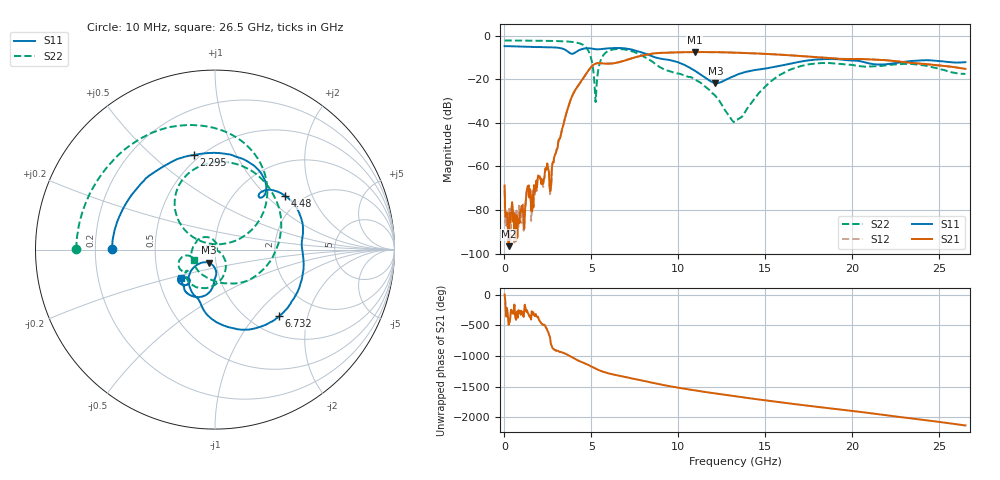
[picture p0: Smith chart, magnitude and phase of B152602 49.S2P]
!  2-Port S-parameters saved by WinCal
! VAR MeasName=S-Parameters (CALIBRATED_DATA) read from VNA (N5242A)
! VAR MeasDate=2016-1-5 16:33:10
! VAR NAME=B152602 49
! VAR FILENAME=B152602 49.S2P
! VAR DATE=2016-1-5 16:33:10
! VAR PHYS_PORTS=1,2
# Hz S DB R 50
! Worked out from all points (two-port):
!   801 points, 10 MHz to 26.5 GHz, reference 50 ohm
!   highest |S21| = -7.55 dB at 10.94 GHz (marker M1); lowest = -96.6 dB at 241.8 MHz (marker M2)
!   |S21| within 3 dB of the highest: 7.255 GHz to 19.01 GHz (11.75 GHz wide, 89.5 % of centre)
!   lowest |S11| = -22.0 dB at 12.13 GHz (marker M3), VSWR 1.17, Z = 46.2 - j6.69 ohm
!   |S11| at or under -10 dB: 8.666 GHz to end of sweep
!   |S22| runs from -39.7 to -2.2 dB; largest |S21 - S12| = 0.0033
!   S11 on the Smith chart (normalised r, x): 10 MHz: 0.27, +0.00; 2.295 GHz: 0.46, +0.69; 4.48 GHz: 1.65, +1.30; 6.732 GHz: 1.33, -1.35; 26.5 GHz: 0.65, -0.22
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1e7  -4.84 179.6  -68.82 2.0  -70.89 131.2  -2.24 179.8
2.417875e8  -4.87 171.4  -96.63 -131.8  -84.56 13.4  -2.25 176.3
1.0696e9  -5.13 144.0  -80.96 26.6  -77.48 56.6  -2.30 163.4
1.367612e9  -5.14 134.3  -69.02 54.5  -71.22 52.1  -2.32 158.7
2.294762e9  -5.34 102.4  -65.51 -130.5  -64.95 -136.9  -2.42 143.0
2.692112e9  -5.37 87.9  -67.46 -100.2  -68.45 -96.1  -2.46 135.4
3.685488e9  -7.58 47.9  -32.31 92.2  -32.31 92.2  -2.75 110.7
4.447075e9  -6.22 38.9  -20.59 -20.2  -20.59 -20.1  -3.95 78.8
4.480188e9  -6.15 37.4  -20.22 -24.2  -20.22 -24.0  -4.08 76.7
4.91065e9  -5.85 17.7  -15.13 -78.2  -15.13 -78.1  -8.54 41.1
5.241775e9  -6.26 5.7  -12.86 -126.5  -12.86 -126.3  -30.52 94.4
5.70535e9  -6.05 -7.7  -12.82 -179.8  -12.82 -179.6  -8.80 127.9
6.731838e9  -5.75 -46.0  -11.90 109.7  -11.88 109.9  -6.21 71.2
7.6921e9  -7.26 -81.4  -9.57 51.1  -9.53 51.2  -8.34 16.3
8.851038e9  -10.41 -106.4  -8.01 -17.8  -7.97 -17.8  -14.05 -71.5
1.093712e10  -16.11 -139.8  -7.55 -120.3  -7.55 -120.3  -20.03 138.4
1.212918e10  -21.96 -115.7  -7.59 -171.3  -7.60 -171.2  -27.66 85.4
1.3255e10  -18.37 -87.2  -7.85 143.1  -7.84 143.1  -39.39 -2.7
1.557288e10  -14.28 -92.3  -8.63 55.8  -8.61 55.6  -19.47 -55.5
1.769208e10  -11.17 -107.2  -9.77 -19.4  -9.73 -19.2  -12.99 -106.7
2.209604e10  -13.00 -128.6  -11.45 -171.2  -11.40 -171.4  -13.53 -143.8
2.65e10  -12.19 -139.6  -15.28 27.7  -15.27 27.6  -17.61 -155.2
